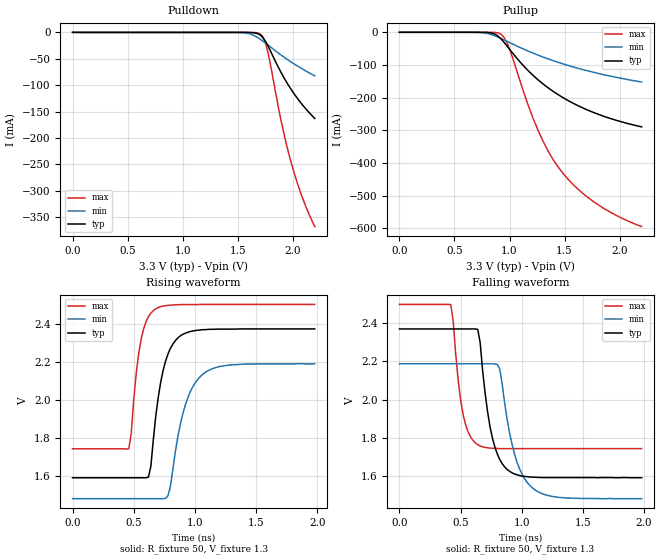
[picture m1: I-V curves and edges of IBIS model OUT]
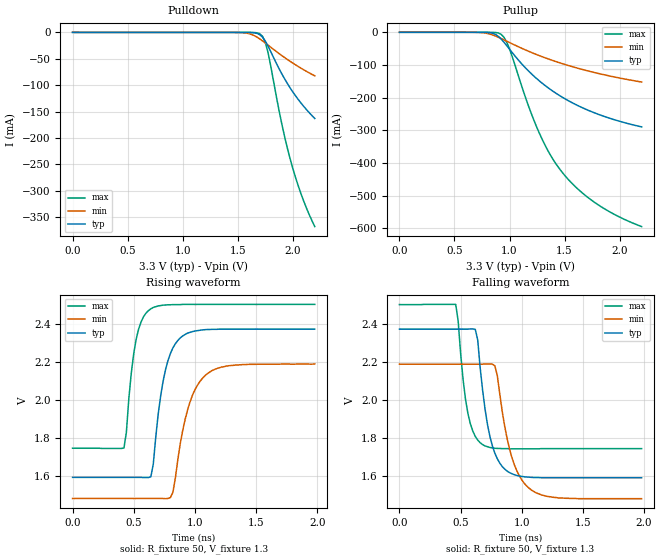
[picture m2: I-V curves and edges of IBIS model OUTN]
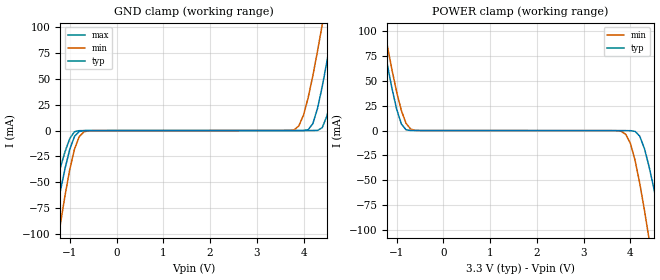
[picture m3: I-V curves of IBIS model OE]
| IBIS file vg4513cb.ibs
| SEIKO EPSON Corp. 2014
[IBIS Ver]   3.2
[File name]   vg4513cb.ibs
[File Rev]   1.0
[Date]   2014/06/30 0:28:33
[Source]
[Notes]
[Disclaimer]
Seiko Epson Corporation makes no warranty with respect to the information
contained herein.
|   vg4513cb
[Component]   VG-4513CB
[Manufacturer]   Seiko Epson Corporation
[Package]
R_pkg   0.36   NA   NA
L_pkg   4.00n   NA   NA
C_pkg   0.42p   NA   NA
[Pin] signal_name   model_name   R_pin   L_pin   C_pin
1   VC   NC
2   OE   OE   0.10   2.00n   0.77p
3   GND   GND
4   OUT   OUT   0.43   4.00n   0.47p
5   OUTN   OUTN   0.28   4.00n   0.38p
6   VCC   POWER
[Diff Pin] inv_pin vdiff   tdelay_typ
4   5   0   0
| Models and submodels in the file (3): OUT (Output_ECL), OUTN (Output_ECL), OE (Input)
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|   Model OUT
[Model]   OUT
Model_type Output_ECL
Enable Active-High
Polarity Non-Inverting
Vref=1.3
Vmeas=1.982
Rref=50
Cref=0
C_comp   0.1p   0.1p   0.1p
[Temperature Range] 25   110   -40
[Voltage Range]   3.3   3.135   3.465
[Pullup Reference]  3.3   3.135   3.465
[Pulldown Reference]3.3   3.135   3.465
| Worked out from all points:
|   falling waveform, R_fixture 50, V_fixture 1.3: 20-80 % time 111ps typ, 146ps min, 84ps max; typ from 2.37 V to 1.59 V
|   rising waveform, R_fixture 50, V_fixture 1.3: 20-80 % time 113ps typ, 149ps min, 84.4ps max; typ from 1.59 V to 2.37 V
[Pullup]
0V        109.6pA    1.947nA    59.12pA
800mV     -591.5uA   -3.656mA   -20.64uA
875mV     -6.95mA    -11.77mA   -732.2uA
925mV     -20.96mA   -19.23mA   -6.473mA
1V        -51.65mA   -31.36mA   -50.91mA
1.15V     -110.7mA   -54.7mA    -204.2mA
1.25V     -142.7mA   -68.65mA   -292.4mA
1.35V     -169.6mA   -81.31mA   -362.8mA
1.45V     -192.5mA   -92.77mA   -415.9mA
1.6V      -220.8mA   -108mA     -472.9mA
1.775V    -246.8mA   -123.4mA   -520.8mA
2.2V      -289.3mA   -152.1mA   -594.3mA
[Pulldown]
0V        122.4uA    211.1uA    4.794uA
1.525V    -7.282uA   -320.5uA   -606.9nA
1.625V    -306uA     -3.796mA   -71.84uA
1.7V      -4.268mA   -12.26mA   -2.476mA
1.725V    -8.871mA   -15.98mA   -7.297mA
1.75V     -16.14mA   -19.91mA   -18.42mA
1.775V    -25.6mA    -23.95mA   -37.74mA
1.9V      -78.19mA   -43.75mA   -172.8mA
1.95V     -96.31mA   -51.08mA   -218.2mA
2V        -112.5mA   -58.03mA   -257.1mA
2.1V      -140.1mA   -70.8mA    -319.6mA
2.2V      -162.9mA   -82.28mA   -367.6mA
[Falling Waveform]
R_fixture=50
V_fixture=1.3
V_fixture_min=1.135
V_fixture_max=1.465
0s        2.371V     2.188V     2.5V
420ps     2.371V     2.188V     2.499V
520ps     2.371V     2.188V     1.923V
640ps     2.369V     2.188V     1.763V
740ps     1.859V     2.188V     1.745V
820ps     1.685V     2.161V     1.742V
880ps     1.633V     1.897V     1.742V
980ps     1.601V     1.639V     1.742V
1.12ns    1.591V     1.52V      1.742V
1.98ns    1.589V     1.479V     1.742V
[Rising Waveform]
R_fixture=50
V_fixture=1.3
V_fixture_min=1.135
V_fixture_max=1.465
0s        1.59V      1.48V      1.742V
460ps     1.59V      1.48V      1.743V
560ps     1.59V      1.48V      2.317V
620ps     1.593V     1.48V      2.437V
680ps     1.913V     1.48V      2.479V
740ps     2.154V     1.48V      2.493V
800ps     2.271V     1.545V     2.498V
920ps     2.35V      1.969V     2.501V
1.06ns    2.369V     2.132V     2.502V
1.98ns    2.373V     2.19V      2.502V
[Ramp]
R_load=50
dV/dt_r   4.702e-1/1.123e-10   4.262e-1/1.488e-10   4.568e-1/8.386e-11
dV/dt_f   4.702e-1/1.113e-10   4.262e-1/1.454e-10   4.568e-1/8.411e-11
|[End   OUT
|   Model OUTN
[Model]   OUTN
Model_type Output_ECL
Enable Active-High
Polarity Inverting
Vref=1.3
Vmeas=1.978
Rref=50
Cref=0
C_comp   0.1p   0.1p   0.1p
[Model Spec]
[Temperature Range] 25   110   -40
[Voltage Range]   3.3   3.135   3.465
[Pullup Reference]  3.3   3.135   3.465
[Pulldown Reference]3.3   3.135   3.465
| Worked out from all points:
|   falling waveform, R_fixture 50, V_fixture 1.3: 20-80 % time 112ps typ, 146ps min, 84.3ps max; typ from 2.37 V to 1.59 V
|   rising waveform, R_fixture 50, V_fixture 1.3: 20-80 % time 113ps typ, 149ps min, 84.4ps max; typ from 1.59 V to 2.37 V
[Pullup]
0V        109.6pA    1.951nA    59.12pA
800mV     -591.1uA   -3.655mA   -20.65uA
875mV     -6.947mA   -11.77mA   -732.3uA
925mV     -20.95mA   -19.23mA   -6.474mA
1V        -51.64mA   -31.35mA   -50.92mA
1.15V     -110.7mA   -54.69mA   -204.2mA
1.25V     -142.7mA   -68.65mA   -292.4mA
1.35V     -169.6mA   -81.3mA    -362.8mA
1.45V     -192.5mA   -92.77mA   -415.9mA
1.6V      -220.8mA   -108mA     -472.9mA
1.775V    -246.8mA   -123.3mA   -520.8mA
2.2V      -289.3mA   -152.1mA   -594.3mA
[Pulldown]
0V        122.4uA    211.1uA    4.795uA
1.525V    -7.286uA   -320.7uA   -606.7nA
1.625V    -306.2uA   -3.798mA   -71.83uA
1.7V      -4.27mA    -12.26mA   -2.475mA
1.725V    -8.875mA   -15.98mA   -7.296mA
1.75V     -16.14mA   -19.91mA   -18.42mA
1.775V    -25.6mA    -23.95mA   -37.74mA
1.9V      -78.2mA    -43.75mA   -172.8mA
1.95V     -96.32mA   -51.09mA   -218.2mA
2V        -112.5mA   -58.03mA   -257.1mA
2.1V      -140.1mA   -70.8mA    -319.6mA
2.2V      -162.9mA   -82.28mA   -367.6mA
[Falling Waveform]
R_fixture=50
V_fixture=1.3
V_fixture_min=1.135
V_fixture_max=1.465
0s        2.374V     2.19V      2.503V
460ps     2.374V     2.19V      2.504V
560ps     2.374V     2.19V      1.93V
620ps     2.373V     2.19V      1.81V
680ps     2.053V     2.19V      1.767V
740ps     1.809V     2.191V     1.752V
800ps     1.693V     2.13V      1.747V
920ps     1.614V     1.698V     1.745V
1.06ns    1.596V     1.538V     1.745V
1.98ns    1.593V     1.483V     1.746V
[Rising Waveform]
R_fixture=50
V_fixture=1.3
V_fixture_min=1.135
V_fixture_max=1.465
0s        1.593V     1.482V     1.746V
420ps     1.593V     1.482V     1.747V
520ps     1.593V     1.482V     2.319V
640ps     1.596V     1.482V     2.479V
760ps     2.159V     1.481V     2.499V
820ps     2.273V     1.514V     2.501V
880ps     2.326V     1.769V     2.501V
980ps     2.359V     2.024V     2.502V
1.14ns    2.371V     2.154V     2.502V
1.98ns    2.372V     2.189V     2.502V
[Ramp]
R_load=50
dV/dt_r   4.696E-1/1.133E-10   4.256E-1/1.498E-10   4.556E-1/8.454E-11
dV/dt_f   4.696E-1/1.122E-10   4.256E-1/1.468E-10   4.556E-1/8.469E-11
|[End   OUTN
|   Model OE
[Model]   OE
Model_type Input
Vinh=2.2
Vinl=1.8
C_comp   2p   2p   2p
[Model Spec]
[Temperature Range] 25   110   -40
[Voltage Range]   3.3   3.135   3.465
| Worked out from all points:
|   GND clamp passes 1 mA (typ) near -0.80 V on its own axis
|   POWER clamp passes 1 mA (typ) near -0.80 V on its own axis
[GND Clamp]
-3.3V     -614.5mA   -809.6mA   -431.2mA
-1.6V     -156mA     -216mA     -106mA
-1.4V     -105.4mA   -151mA     -69.78mA
-1.2V     -57.78mA   -89.94mA   -35.51mA
-900mV    -5.677mA   -17.99mA   -1.153mA
-600mV    -82.32uA   -224.5uA   -82.43uA
3.8V      10.34uA    681.1uA    6.789uA
4V        41.56uA    14.86mA    10.84uA
4.3V      21.39mA    76.59mA    91.28uA
4.6V      92.16mA    155.3mA    31.83mA
4.9V      174.6mA    239.2mA    97.17mA
6.6V      675.5mA    740.7mA    510.3mA
[POWER Clamp]
-3.3V     675.5mA    691.2mA    NA
-1.4V     119mA      137.6mA    NA
-1.3V     92.16mA    111mA      NA
-1V       21.39mA    38.75mA    NA
-800mV    783.3uA    7.29mA     NA
3.8V      -78.6uA    -711.9uA   NA
4V        -124.1uA   -12.89mA   NA
4.1V      -863.6uA   -29.89mA   NA
4.2V      -5.677mA   -52.99mA   NA
4.4V      -36.28mA   -109.2mA   NA
4.7V      -105.4mA   -204.4mA   NA
6.6V      -614.5mA   -868.6mA   NA
